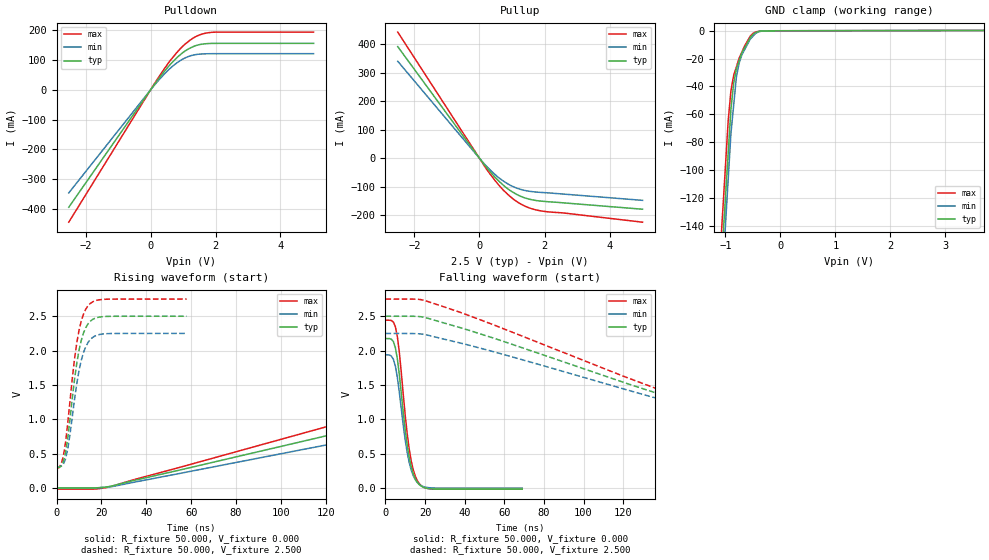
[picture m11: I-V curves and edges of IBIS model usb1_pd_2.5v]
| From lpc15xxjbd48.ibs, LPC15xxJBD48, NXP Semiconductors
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[Model]   usb1_pd_2.5v
Model_type I/O
Vinl=8.000E-01
Vinh=1.750E+00
Vref=0.000E+00
Rref=1.000E+06
Cref=0.000E+00
Vmeas=1.250E+00
C_comp   2.000E-12   2.000E-12   2.000E-12
[Voltage Range]   2.500E+00   2.250E+00   2.750E+00
[POWER Clamp Reference]   2.500E+00   2.250E+00   2.750E+00
[GND Clamp Reference]   0.000E+00   0.000E+00   0.000E+00
[Pullup Reference]   2.500E+00   2.250E+00   2.750E+00
[Pulldown Reference]   0.000E+00   0.000E+00   0.000E+00
[Temperature Range]   25   85   -40
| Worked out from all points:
|   slope of the pulldown table from 0 to 0.375 V, typ, clamps not added: 6.8 ohm
|   slope of the pullup table from 0 to 0.375 V, typ, clamps not added: 6.99 ohm
|   GND clamp passes 1 mA (typ) near -0.43 V on its own axis
|   rising waveform, R_fixture 50.000, V_fixture 0.000: 20-80 % time 190ns typ, 204ns min, 177ns max; typ from 0 V to 2.2 V
|   falling waveform, R_fixture 50.000, V_fixture 0.000: 20-80 % time 5.54ns typ, 5.62ns min, 5.44ns max; typ from 2.18 V to -0.014 V
|   rising waveform, R_fixture 50.000, V_fixture 2.500: 20-80 % time 5.36ns typ, 5.45ns min, 5.37ns max; typ from 0.301 V to 2.5 V
|   falling waveform, R_fixture 50.000, V_fixture 2.500: 20-80 % time 143ns typ, 150ns min, 137ns max; typ from 2.5 V to 0.301 V
[GND Clamp]
-2.5V     -1.074A    -1.128A    -1.079A
-950mV    -88.11mA   -106.7mA   -64.68mA
-900mV    -56.29mA   -73.73mA   -43.18mA
-850mV    -37.7mA    -53.38mA   -32.03mA
-800mV    -27.09mA   -33.02mA   -25.84mA
-750mV    -21.44mA   -23.17mA   -19.65mA
-700mV    -15.79mA   -17.18mA   -15.24mA
-550mV    -5.066mA   -6.107mA   -4.019mA
-450mV    -1.222mA   -1.839mA   -871.2uA
-350mV    -218.7uA   -361.7uA   -202.2uA
-150mV    -19.54uA   -41.46uA   -18.78uA
5V        297.7uA    308.5uA    296.1uA
[Power Clamp]
-2.51V    0A         0A         0A
0V        0A         0A         0A
2.5V      0A         0A         0A
5V        0A         0A         0A
[Pullup]
-2.51V    392.3mA    340.9mA    443.4mA
230mV     -33.95mA   -29.9mA    -40.38mA
470mV     -65.73mA   -56.29mA   -76.87mA
690mV     -90.27mA   -76.71mA   -106.7mA
1.05V     -121.1mA   -100.7mA   -144.5mA
1.43V     -140.7mA   -114.1mA   -170.1mA
1.85V     -150.2mA   -119.8mA   -184.3mA
5.01V     -179.1mA   -148.1mA   -224.8mA
[Pulldown]
-2.52V    -393.9mA   -345.8mA   -444.1mA
160mV     24.62mA    21.35mA    27.98mA
480mV     69.42mA    59.44mA    79.66mA
740mV     100.4mA    84.72mA    116.4mA
960mV     122.2mA    101.4mA    143.1mA
1.18V     138.2mA    112.6mA    163.8mA
1.5V      151.7mA    119.9mA    184.1mA
1.88V     155.9mA    121.4mA    193mA
5.02V     156.1mA    121.5mA    193.9mA
[Rising Waveform]
R_fixture = 50.000
V_fixture = 0.000
V_fixture_min = 0.000
V_fixture_max = 0.000
|  time   V(typ)   V(min)   V(max)
0s        58.31uV    199.8uV    -15.47mV
23ns      19.65mV    13.15mV    12.49mV
124ns     788.5mV    651mV      925.5mV
194ns     1.294V     1.073V     1.52V
253ns     1.674V     1.393V     1.961V
291ns     1.871V     1.571V     2.169V
338ns     2.022V     1.728V     2.304V
401ns     2.12V      1.841V     2.382V
472ns     2.167V     1.901V     2.418V
586ns     2.197V     1.94V      2.441V
[Falling Waveform]
R_fixture = 50.000
V_fixture = 0.000
V_fixture_min = 0.000
V_fixture_max = 0.000
|  time   V(typ)   V(min)   V(max)
0s        2.176V     1.94V      2.442V
3ns       2.166V     1.92V      2.438V
5ns       2.042V     1.773V     2.348V
7ns       1.648V     1.393V     1.973V
10ns      836.6mV    692.8mV    1.048V
12ns      445mV      371.3mV    563.7mV
14ns      211.7mV    183mV      269mV
17ns      53.51mV    56.11mV    67.14mV
24ns      -11.07mV   2.623mV    -12.71mV
69ns      -13.61mV   199.8uV    -14.78mV
[Rising Waveform]
R_fixture = 50.000
V_fixture = 2.500
V_fixture_min = 2.250
V_fixture_max = 2.750
|  time   V(typ)   V(min)   V(max)
0s        301.1mV    307.8mV    293.6mV
2ns       319.4mV    314.6mV    344.4mV
3ns       378.4mV    343.9mV    455.6mV
4ns       512.9mV    421.8mV    658.3mV
6ns       1.006V     780.7mV    1.267V
9ns       1.811V     1.514V     2.108V
11ns      2.147V     1.856V     2.429V
14ns      2.388V     2.117V     2.651V
21ns      2.495V     2.243V     2.746V
58ns      2.5V       2.25V      2.75V
[Falling Waveform]
R_fixture = 50.000
V_fixture = 2.500
V_fixture_min = 2.250
V_fixture_max = 2.750
|  time   V(typ)   V(min)   V(max)
0s        2.5V       2.25V      2.75V
17ns      2.496V     2.244V     2.745V
31ns      2.39V      2.157V     2.623V
165ns     1.126V     1.091V     1.149V
210ns     740.3mV    762.6mV    703.4mV
233ns     570.3mV    612.1mV    520.4mV
259ns     443.1mV    482.3mV    404.8mV
292ns     365.9mV    390.3mV    342mV
334ns     323.3mV    336.5mV    310.2mV
393ns     301.1mV    307.8mV    293.6mV
[Ramp]
dV/dt_r   1.3136E+00/1.8912E-07   1.1585E+00/2.0389E-07   1.4741E+00/1.7664E-07
dV/dt_f   1.3193E+00/1.4271E-07   1.1653E+00/1.4991E-07   1.4738E+00/1.3645E-07
R_load = 50
